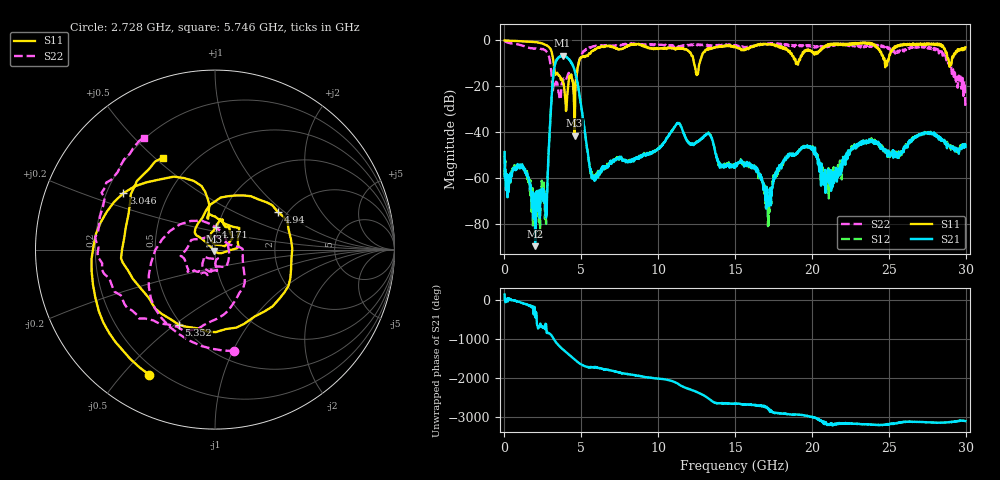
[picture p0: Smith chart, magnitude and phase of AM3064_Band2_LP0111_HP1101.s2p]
# Hz S DB R 50.0
!freq dBS11 angS11 dBS21 angS21 dBS12 angS12 dBS22 angS22
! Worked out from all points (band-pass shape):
!   1600 points, 10 MHz to 29.98 GHz, reference 50 ohm
!   highest |S21| = -6.70 dB at 3.777 GHz (marker M1); lowest = -89.5 dB at 1.997 GHz (marker M2)
!   |S21| within 3 dB of the highest: 3.317 GHz to 4.338 GHz (1.021 GHz wide, 26.7 % of centre); 4.349085 GHz to 4.361086 GHz (12 MHz wide, 0.276 % of centre)
!   lowest |S11| = -41.4 dB at 4.565 GHz (marker M3), VSWR 1.02, Z = 49.7 - j0.803 ohm
!   |S11| at or under -10 dB: 3.202 GHz to 4.822 GHz (1.62 GHz wide, 40.4 % of centre); 12.33 GHz to 12.69 GHz (351.1 MHz wide, 2.81 % of centre); 28.91 GHz to 29.08 GHz (165.8 MHz wide, 0.572 % of centre)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
!   |S22| runs from -29.2 to -0.3 dB; largest |S21 - S12| = 0.012
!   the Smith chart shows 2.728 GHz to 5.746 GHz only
!   S11 on the Smith chart (normalised r, x): 2.728 GHz: 0.16, -0.59; 3.046 GHz: 0.27, +0.26; 4.171 GHz: 0.97, +0.25; 4.94 GHz: 1.79, +0.90; 5.352 GHz: 0.48, -0.52; 5.746 GHz: 0.34, +0.53
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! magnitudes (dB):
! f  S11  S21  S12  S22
! 10 MHz  0.0  -48.5  -49.9  -0.3
! 1.322 GHz  -0.5  -56.0  -55.4  -2.7
! 1.997 GHz  -0.7  -89.5  -78.6  -3.6
! 2.728 GHz  -2.1  -74.6  -75.2  -4.8
! 3.046 GHz  -4.4  -26.9  -26.9  -13.6
! 3.777 GHz  -17.9  -6.7  -6.8  -18.7
! 4.171 GHz  -17.9  -8.1  -8.0  -14.1
! 4.565 GHz  -41.4  -13.0  -12.9  -23.4
! 4.94 GHz  -7.8  -26.6  -26.5  -7.0
! 5.015 GHz  -7.4  -29.8  -29.7  -6.4
! 5.352 GHz  -6.6  -45.6  -46.0  -3.7
! 5.746 GHz  -4.6  -59.5  -59.3  -2.6
! 10 GHz  -3.6  -47.2  -46.7  -1.9
! 11.31 GHz  -3.2  -36.2  -35.9  -2.6
! 15 GHz  -2.7  -54.4  -54.4  -2.1
! 17.12 GHz  -1.7  -71.9  -74.2  -1.4
! 19.99 GHz  -4.6  -47.0  -46.4  -2.2
! 21.17 GHz  -1.9  -57.5  -62.0  -1.9
! 23.2 GHz  -1.2  -45.4  -45.2  -2.3
! 25 GHz  -8.2  -49.7  -50.2  -3.1
! 28.31 GHz  -2.1  -42.1  -42.6  -4.7
! 29.98 GHz  -3.0  -46.3  -46.7  -29.2
